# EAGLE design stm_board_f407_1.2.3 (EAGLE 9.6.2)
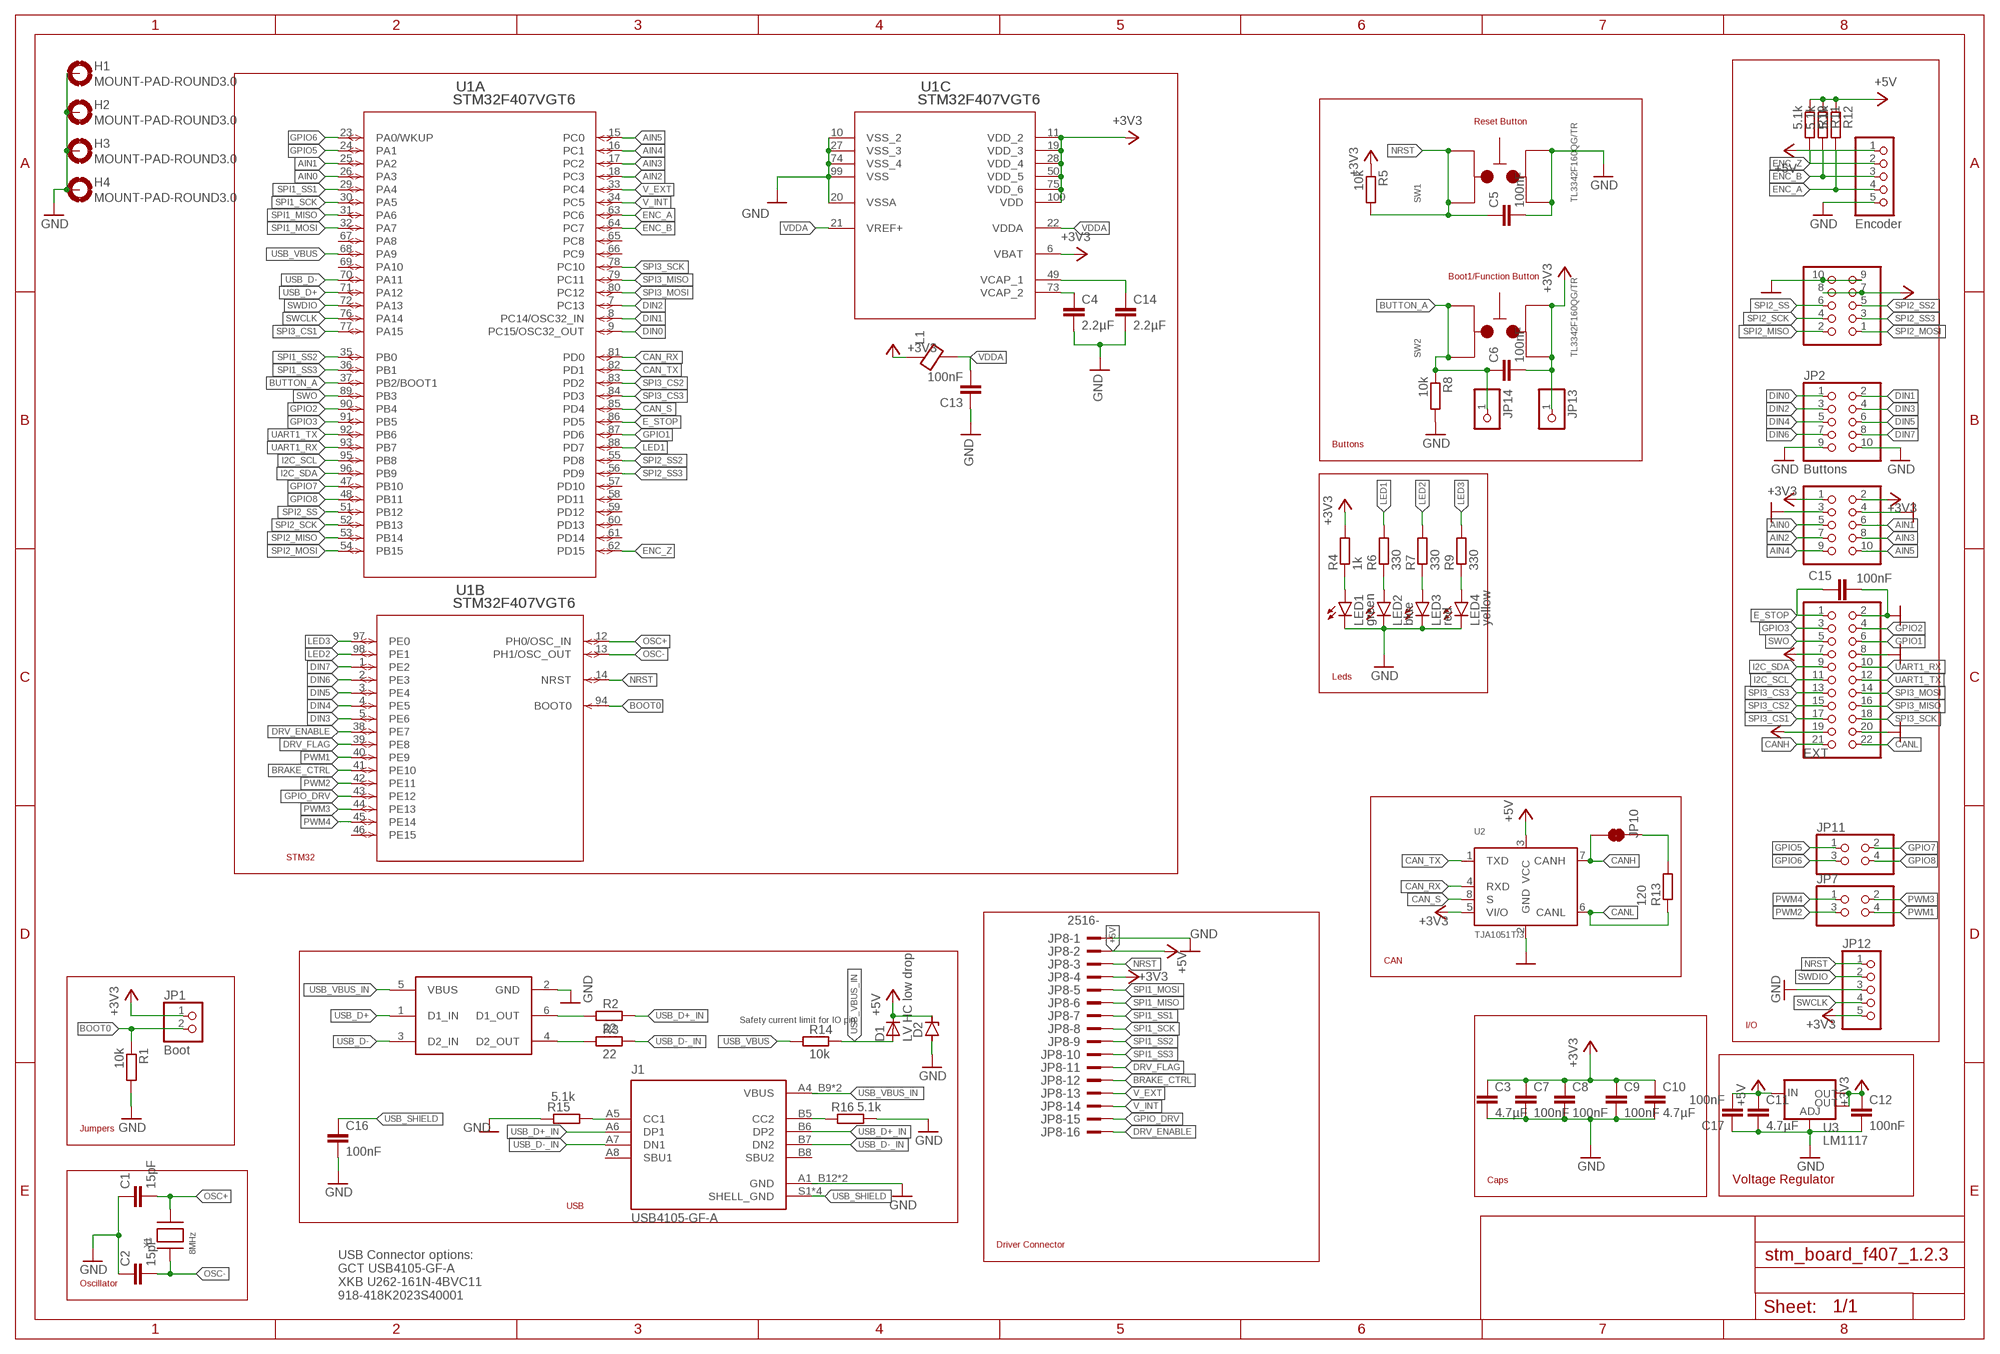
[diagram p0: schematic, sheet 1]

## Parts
C1  15pF  C-EUC0603  [C0603]
C2  15pF  C-EUC0603  [C0603]
C3  4.7µF  C-EUC0805  [C0805]
C4  2.2µF  C-EUC0603  [C0603]
C5  100nF  C-EUC0603  [C0603]
C6  100nF  C-EUC0603  [C0603]
C7  100nF  C-EUC0603  [C0603]
C8  100nF  C-EUC0603  [C0603]
C9  100nF  C-EUC0603  [C0603]
C10  4.7µF  C-EUC0805  [C0805]
C11  4.7µF  C-EUC0805  [C0805]
C12  100nF  C-EUC0603  [C0603]
C13  100nF  C-EUC0603  [C0603]
C14  2.2µF  C-EUC0603  [C0603]
C15  100nF  C-EUC0603  [C0603]
C16  100nF  C-EUC0603  [C0603]
C17  100nF  C-EUC0603  [C0603]
D1  LV HC low drop  DIODESMA  [SMADIODE]
D2  ZENER-DIODESOD80C  [SOD80C]
H1  MOUNT-PAD-ROUND3.0  [3,0-PAD]
H2  MOUNT-PAD-ROUND3.0  [3,0-PAD]
H3  MOUNT-PAD-ROUND3.0  [3,0-PAD]
H4  MOUNT-PAD-ROUND3.0  [3,0-PAD]
J1  USB4105-GF-A  [GCT_USB4105-GF-A]
JP1  Boot  PINHD-1X2  [1X02]
JP2  Buttons  PINHD-2X5  [2X05]
JP3  Analog  PINHD-2X5  [2X05]
JP4  EXT  PINHD-2X11  [2X11]
JP5  Encoder  PINHD-1X5  [1X05]
JP6  SPI  PINHD-2X5  [2X05]
JP7  PINHD-2X2  [2X02]
JP8  2516-  [PAK100/2500-16]
JP10  JUMPER-SMT_2_NC_TRACE_SILK  [SMT-JUMPER_2_NC_TRACE_SILK]
JP11  PINHD-2X2  [2X02]
JP12  PINHD-1X5  [1X05]
JP13  PINHD-1X1  [1X01]
JP14  PINHD-1X1  [1X01]
L1  GZ2012D601TF  BLM21PG331SN1D  [BLM21PG331SN1D]
LED1  green  LEDSML0805  [SML0805]
LED2  blue  LEDSML0805  [SML0805]
LED3  red  LEDSML0805  [SML0805]
LED4  yellow  LEDSML0805  [SML0805]
R1  10k  R-EU_R0603  [R0603]
R2  22  R-EU_R0603  [R0603]
R3  22  R-EU_R0603  [R0603]
R4  1k  R-EU_R0603  [R0603]
R5  10k  R-EU_R0603  [R0603]
R6  330  R-EU_R0603  [R0603]
R7  330  R-EU_R0603  [R0603]
R8  10k  R-EU_R0603  [R0603]
R9  330  R-EU_R0603  [R0603]
R10  5.1k  R-EU_R0603  [R0603]
R11  5.1k  R-EU_R0603  [R0603]
R12  5.1k  R-EU_R0603  [R0603]
R13  120  R-EU_R0603  [R0603]
R14  10k  R-EU_R0603  [R0603]
R15  5.1k  R-EU_R0603  [R0603]
R16  5.1k  R-EU_R0603  [R0603]
SW1  TL3342F160QG/TR  [TL3342F160QG/TR]
SW2  TL3342F160QG/TR  [TL3342F160QG/TR]
U1  STM32F407VGT6  [LQFP100-14X14MM]
U2  TJA1051T/3  [SOT96-1]
U3  LM1117  V_REG_LM1117SOT223  [SOT223]
U4  USBLC6-2SC6  [TSOT-23-6]
X1  8MHz  XTALNX5032  [NX5032]

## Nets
+3V3: C3.1 C6.2 C7.1 C8.1 C9.1 C10.1 C12.1 JP1.1 JP3.1 JP3.2 JP4.7 JP6.7 JP6.8 JP8.4 JP12.5 JP13.1 L1.1 R4.2 R5.1 SW2.1 SW2.2 U1.6(C:VBAT) U1.11(C:VDD_2) U1.19(C:VDD_3) U1.28(C:VDD_4) U1.50(C:VDD_5) U1.75(C:VDD_6) U1.100(C:VDD) U2.5(VI/O) U3.2(OUT) U3.4(OUT)
+5V: C11.1 C17.2 D1.C D2.C JP4.19 JP5.1 JP8.2 R10.1 R11.1 R12.1 U2.3(VCC) U3.3(IN)
AIN0: JP3.5 U1.26(A:PA3)
AIN1: JP3.6 U1.25(A:PA2)
AIN2: JP3.7 U1.18(A:PC3)
AIN3: JP3.8 U1.17(A:PC2)
AIN4: JP3.9 U1.16(A:PC1)
AIN5: JP3.10 U1.15(A:PC0)
BOOT0: JP1.2 R1.1 U1.94(B:BOOT0)
BRAKE_CTRL: JP8.12 U1.41(B:PE10)
BUTTON_A: C6.1 JP14.1 R8.1 SW2.3 SW2.4 U1.37(A:PB2/BOOT1)
CAN_RX: U1.81(A:PD0) U2.4(RXD)
CAN_S: U1.85(A:PD4) U2.8(S)
CAN_TX: U1.82(A:PD1) U2.1(TXD)
CANH: JP4.21 JP10.2 U2.7(CANH)
CANL: JP4.22 R13.1 U2.6(CANL)
DIN0: JP2.1 U1.9(A:PC15/OSC32_OUT)
DIN1: JP2.2 U1.8(A:PC14/OSC32_IN)
DIN2: JP2.3 U1.7(A:PC13)
DIN3: JP2.4 U1.5(B:PE6)
DIN4: JP2.5 U1.4(B:PE5)
DIN5: JP2.6 U1.3(B:PE4)
DIN6: JP2.7 U1.2(B:PE3)
DIN7: JP2.8 U1.1(B:PE2)
DRV_ENABLE: JP8.16 U1.38(B:PE7)
DRV_FLAG: JP8.11 U1.39(B:PE8)
E_STOP: C15.1 JP4.1 U1.86(A:PD5)
ENC_A: JP5.4 R12.2 U1.63(A:PC6)
ENC_B: JP5.3 R11.2 U1.64(A:PC7)
ENC_Z: JP5.2 R10.2 U1.62(A:PD15)
GND: C1.1 C2.1 C3.2 C4.2 C5.2 C7.2 C8.2 C9.2 C10.2 C11.2 C12.2 C13.1 C14.2 C15.2 C16.2 C17.1 D2.A H1.B3,0(MOUNT) H2.B3,0(MOUNT) H3.B3,0(MOUNT) H4.B3,0(MOUNT) J1.A1_B12(GND) J1.B1_A12(GND) JP2.9 JP2.10 JP3.3 JP3.4 JP4.2 JP4.8 JP4.20 JP5.5 JP6.9 JP6.10 JP8.1 JP12.3 LED1.C LED2.C LED3.C LED4.C R1.2 R8.2 R15.1 R16.2 SW1.1 SW1.2 U1.10(C:VSS_2) U1.20(C:VSSA) U1.27(C:VSS_3) U1.74(C:VSS_4) U1.99(C:VSS) U2.2(GND) U3.1(ADJ) U4.2(GND)
GPIO1: JP4.6 U1.87(A:PD6)
GPIO2: JP4.4 U1.90(A:PB4)
GPIO3: JP4.3 U1.91(A:PB5)
GPIO5: JP11.1 U1.24(A:PA1)
GPIO6: JP11.3 U1.23(A:PA0/WKUP)
GPIO7: JP11.2 U1.47(A:PB10)
GPIO8: JP11.4 U1.48(A:PB11)
GPIO_DRV: JP8.15 U1.43(B:PE12)
I2C_SCL: JP4.11 U1.95(A:PB8)
I2C_SDA: JP4.9 U1.96(A:PB9)
LED1: R6.2 U1.88(A:PD7)
LED2: R7.2 U1.98(B:PE1)
LED3: R9.2 U1.97(B:PE0)
N$1: R2.1 U4.6(D1_OUT)
N$2: LED4.A R9.1
N$3: JP10.1 R13.2
N$4: C14.1 U1.49(C:VCAP_1)
N$5: J1.B5(CC2) R16.1
N$6: J1.A5(CC1) R15.2
N$7: C4.1 U1.73(C:VCAP_2)
N$8: R3.1 U4.4(D2_OUT)
N$11: LED1.A R4.1
N$12: LED2.A R6.1
N$13: LED3.A R7.1
NRST: C5.1 JP8.3 JP12.1 R5.2 SW1.3 SW1.4 U1.14(B:NRST)
OSC+: C1.2 U1.12(B:PH0/OSC_IN) X1.P$2
OSC-: C2.2 U1.13(B:PH1/OSC_OUT) X1.P$1
PWM1: JP7.4 U1.40(B:PE9)
PWM2: JP7.3 U1.42(B:PE11)
PWM3: JP7.2 U1.44(B:PE13)
PWM4: JP7.1 U1.45(B:PE14)
SPI1_MISO: JP8.6 U1.31(A:PA6)
SPI1_MOSI: JP8.5 U1.32(A:PA7)
SPI1_SCK: JP8.8 U1.30(A:PA5)
SPI1_SS1: JP8.7 U1.29(A:PA4)
SPI1_SS2: JP8.9 U1.35(A:PB0)
SPI1_SS3: JP8.10 U1.36(A:PB1)
SPI2_MISO: JP6.2 U1.53(A:PB14)
SPI2_MOSI: JP6.1 U1.54(A:PB15)
SPI2_SCK: JP6.4 U1.52(A:PB13)
SPI2_SS: JP6.6 U1.51(A:PB12)
SPI2_SS2: JP6.5 U1.55(A:PD8)
SPI2_SS3: JP6.3 U1.56(A:PD9)
SPI3_CS1: JP4.17 U1.77(A:PA15)
SPI3_CS2: JP4.15 U1.83(A:PD2)
SPI3_CS3: JP4.13 U1.84(A:PD3)
SPI3_MISO: JP4.16 U1.79(A:PC11)
SPI3_MOSI: JP4.14 U1.80(A:PC12)
SPI3_SCK: JP4.18 U1.78(A:PC10)
SWCLK: JP12.4 U1.76(A:PA14)
SWDIO: JP12.2 U1.72(A:PA13)
SWO: JP4.5 U1.89(A:PB3)
UART1_RX: JP4.10 U1.93(A:PB7)
UART1_TX: JP4.12 U1.92(A:PB6)
USB_D+: U1.71(A:PA12) U4.1(D1_IN)
USB_D+_IN: J1.A6(DP1) J1.B6(DP2) R2.2
USB_D-: U1.70(A:PA11) U4.3(D2_IN)
USB_D-_IN: J1.A7(DN1) J1.B7(DN2) R3.2
USB_SHIELD: C16.1 J1.S1(SHELL_GND) J1.S2(SHELL_GND) J1.S3(SHELL_GND) J1.S4(SHELL_GND)
USB_VBUS: R14.1 U1.68(A:PA9)
USB_VBUS_IN: D1.A J1.A4_B9(VBUS) J1.B4_A9(VBUS) R14.2 U4.5(VBUS)
V_EXT: JP8.13 U1.33(A:PC4)
V_INT: JP8.14 U1.34(A:PC5)
VDDA: C13.2 L1.2 U1.21(C:VREF+) U1.22(C:VDDA)
Unconnected: J1.A8(SBU1) J1.B8(SBU2) U1.46(B:PE15) U1.57(A:PD10) U1.58(A:PD11) U1.59(A:PD12) U1.60(A:PD13) U1.61(A:PD14) U1.65(A:PC8) U1.66(A:PC9) U1.67(A:PA8) U1.69(A:PA10)

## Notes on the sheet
- Reset Button
- Boot1/Function Button
- Buttons
- Leds
- STM32
- CAN
- Safety current limit for IO pin
- I/O
- Jumpers
- Caps | Voltage Regulator
- USB
- Driver Connector
- Oscillator
- USB Connector options:
  GCT USB4105-GF-A 
  XKB U262-161N-4BVC11
  918-418K2023S40001

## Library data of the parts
C1-C17 = resistor:C-EU: CAPACITOR, European symbol
D1 = adafruit:DIODE: Diode
D2 = diode:ZENER-DIODE: Z-Diode
H1-H4 = holes:MOUNT-PAD-ROUND: MOUNTING PAD, round
J1 = USB4105-GF-A:USB4105-GF-A: USB-C (USB TYPE-C) USB 2.0 Receptacle Connector 24 (16+8 Dummy) Position Surface Mount, Right Angle; Through Hole Check availability; AVAILABILITY: In Stock; DESCRIPTION: USB-C (USB TYPE-C) USB 2.0 Receptacle Connector 24 (16+8 Dummy) Position Surface Mount, Right Angle; Through Hole; MF: GCT; MP: USB4105-GF-A; PACKAGE: None; PRICE: None; PURCHASE-URL: https://pricing.snapeda.com/search/part/USB4105-GF-A/?ref=eda
JP1 = pinhead:PINHD-1X2: PIN HEADER
JP2 JP3 JP6 = pinhead:PINHD-2X5: PIN HEADER
JP4 = pinhead:PINHD-2X11: PIN HEADER
JP5 JP12 = pinhead:PINHD-1X5: PIN HEADER
JP7 JP11 = pinhead:PINHD-2X2: PIN HEADER
JP8 = con-3m:2516-: 3M (TM) Pak 100 4-Wall Header Source: 3M; OC_FARNELL: unknown; OC_NEWARK: unknown
JP10 = SparkFun-Jumpers:JUMPER-SMT_2_NC_TRACE: Normally closed trace jumper
JP13 JP14 = pinhead:PINHD-1X1: PIN HEADER
L1 = Thermistor_Inductors:BLM21PG331SN1D: FERRITE BEAD 330 OHM 0805 1LN; CREATED_BY: PCBLayout.com; DIGIKEY_PART_NUMBER: 490-5988-2-ND; MANUFACTURER: Murata Electronics North America; MPN: BLM21PG331SN1D; PACKAGE: 0805
LED1-LED4 = led:LED: LED
R1-R16 = resistor:R-EU_: RESISTOR, European symbol
SW1 SW2 = Switch:TL3342F160QG/TR: SWITCH TACTILE SPST-NO 0.05A 12V Manufacturer's datasheet; CREATED_BY: PCBLayout.com; DIGI_KEY_PART_NUMBER: EG2531CT-ND; MANUFACTURER: E-Switch; MPN: TL3342F160QG/TR; PACKAGE: SPST_NO
U1 = STM32:STM32F407VGT6; BUILT_BY: EMA_UL_Team; COPYRIGHT: Copyright (C) 2018 Accelerated Designs. All rights reserved; MANUFACTURER_PART_NUMBER: STM32F407VGT6; SOURCELIBRARY: Updates_to_database_2020-10-19; VENDOR: STMicroelectronics
U2 = TJA1051T_3:TJA1051T/3: High-speed CAN transceiver The TJA1051 is a high-speed CAN transceiver that provides an interface between a Controller Area Network (CAN) protocol controller and the physical two-wire CAN bus. The transceiver is designed for high-speed (up to 1 Mbit/s) CAN applications in the automotive industry,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; AVAILABILITY: Bad; DESCRIPTION: 1/1 Transceiver Half CANbus 8-SO; MF: NXP Semiconductors; MP: TJA1051T/3; PACKAGE: SOIC-8 NXP Semiconductors; PRICE: None
U3 = SparkFun-IC-Power:V_REG_LM1117: Voltage Regulator LM1117 Standard adjustable voltage regulator but in SMD form. Spark Fun Electronics SKU : COM-00595; PROD_ID: VREG-08170
U4 = con_ampusb_10118193-0001LF:USBLC6-2SC6
X1 = adafruit:XTAL: Low cost SMT crystals, no capacitors included

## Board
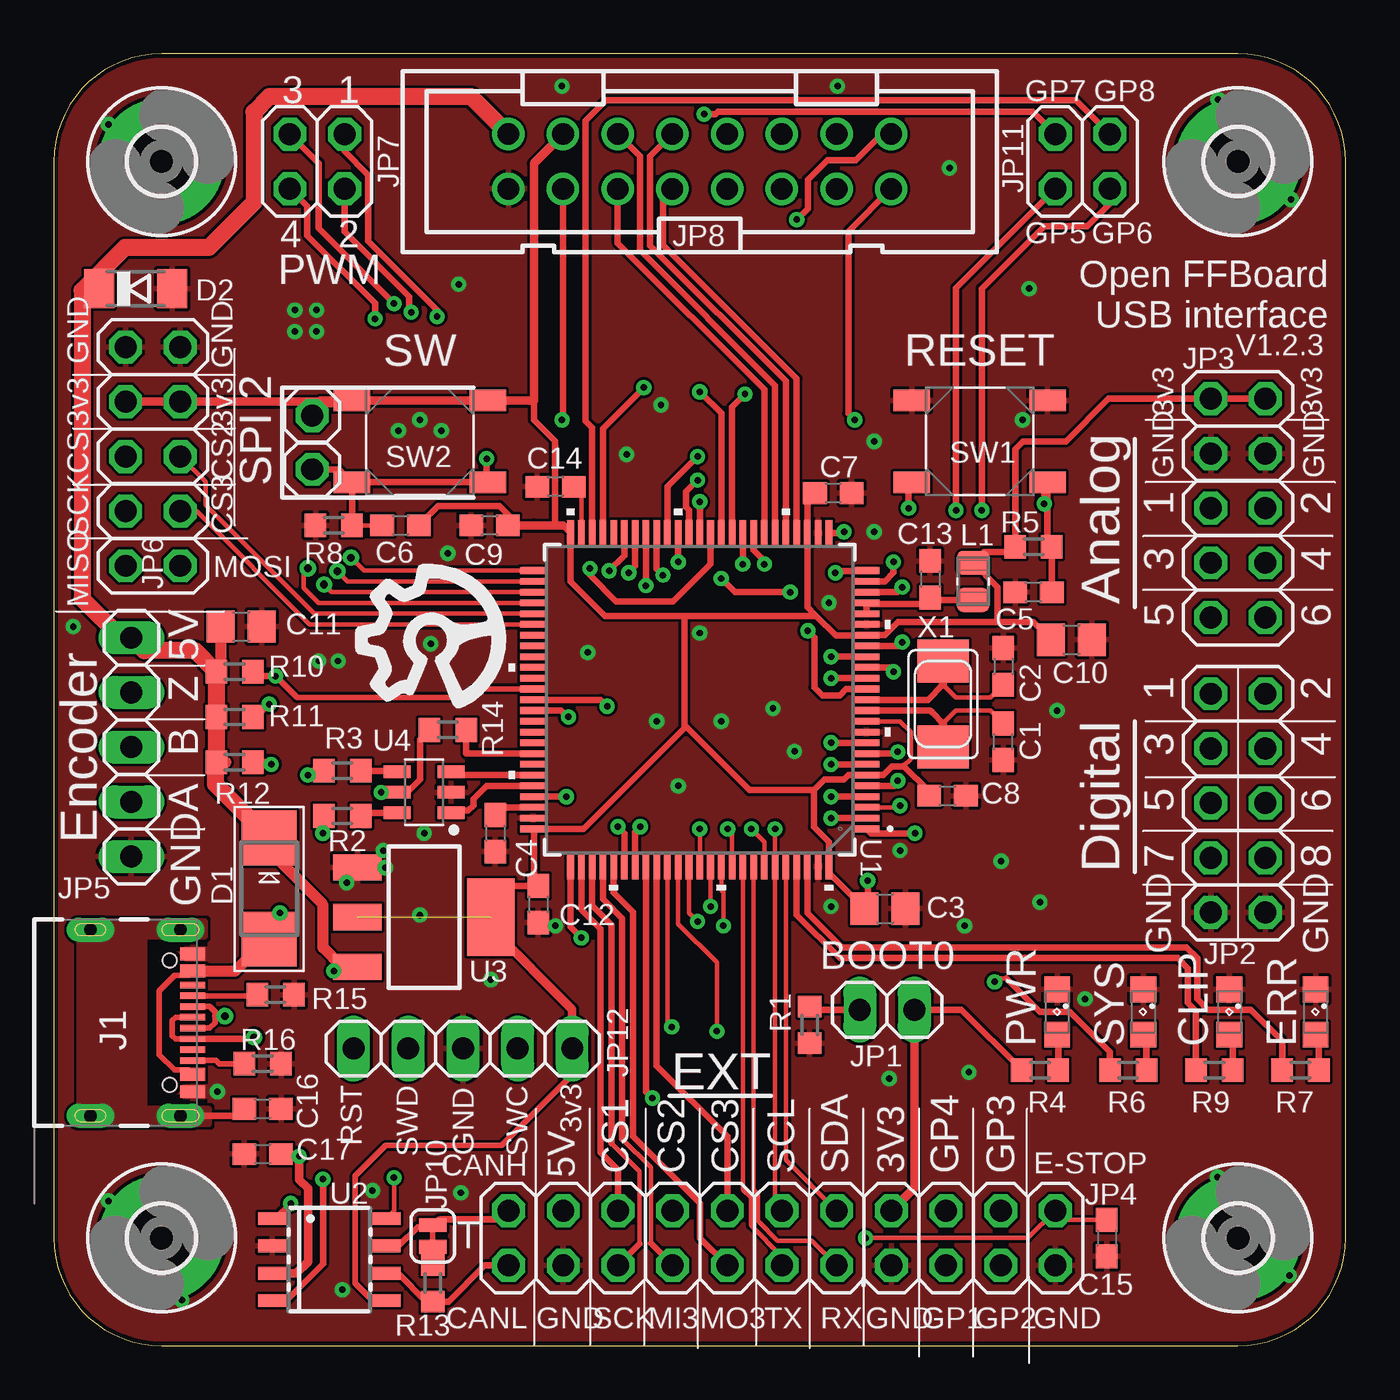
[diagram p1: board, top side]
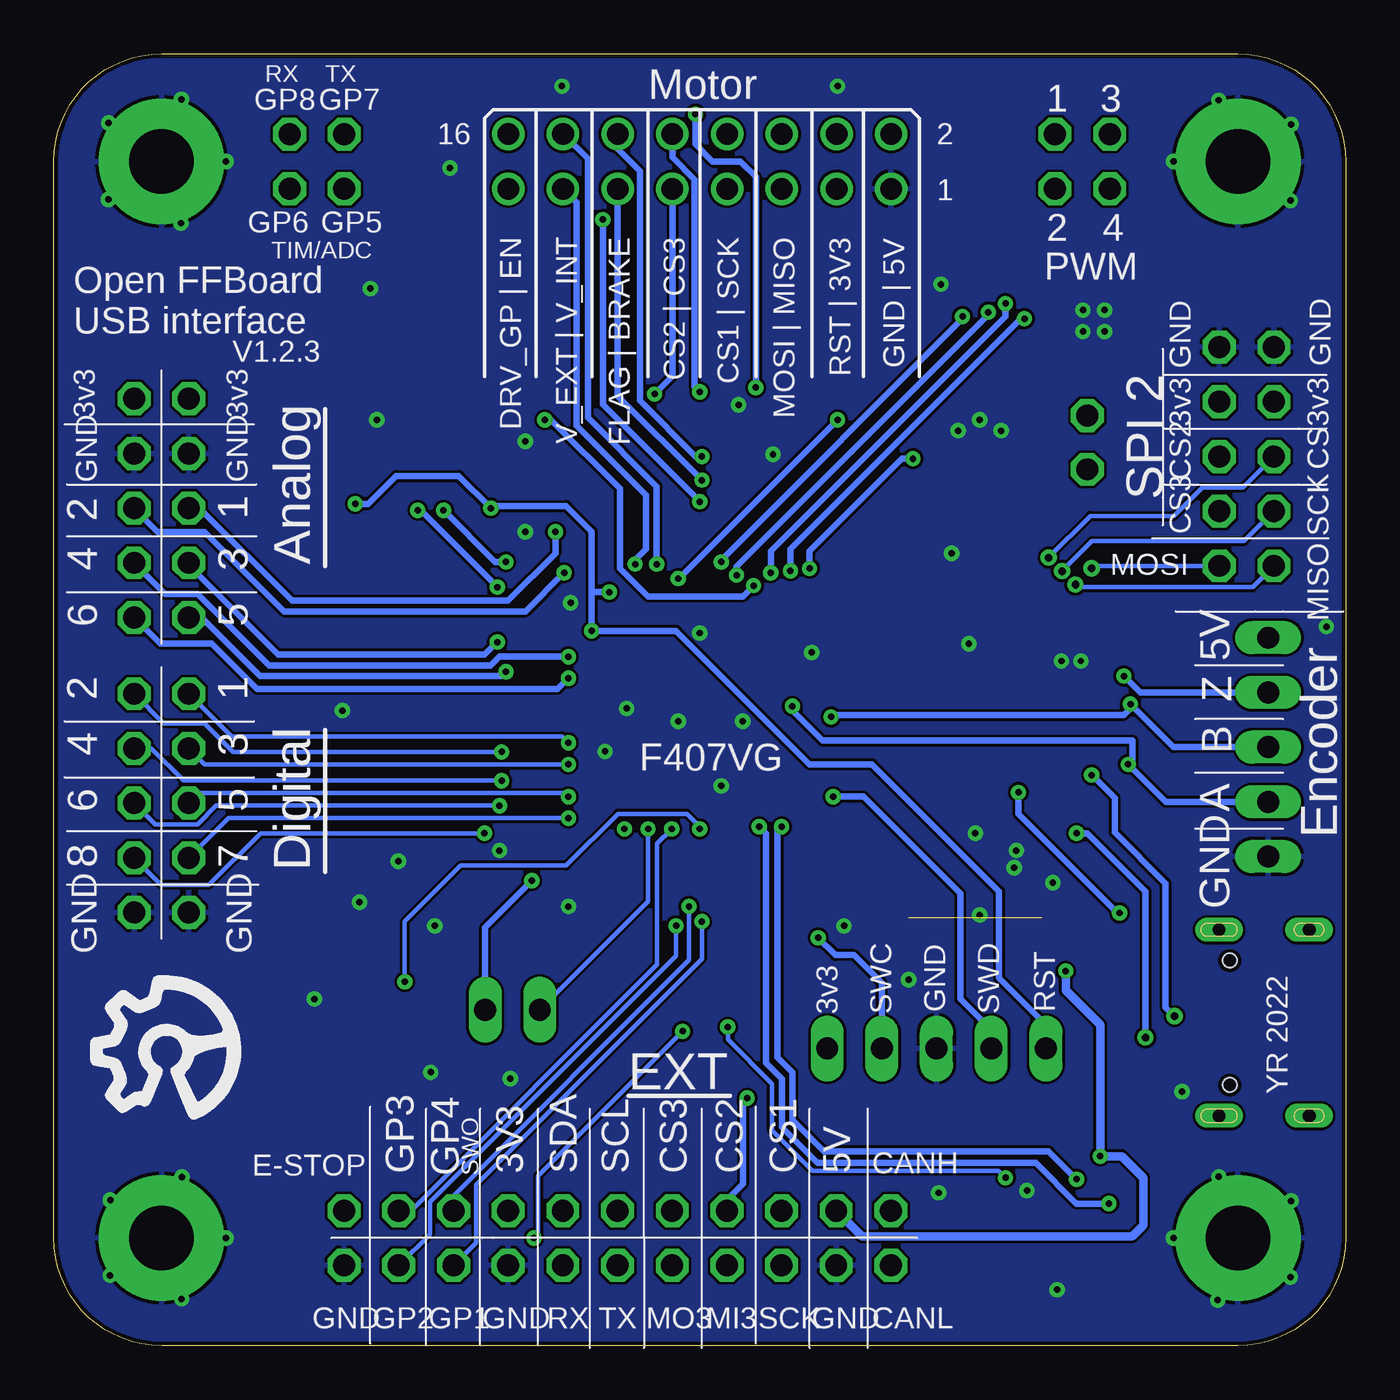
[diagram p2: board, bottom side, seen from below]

Size 60 x 60 mm. Coordinates in mm from the lower left corner, seen from the top.
Outline: 5,0 55,0 arc90 60,5 60,55 arc90 55,60 5,60 arc90 0,55 0,5 arc90 5,0
Copper layers (1*16): Top 0.035mm / dielectric 1.5mm / Bottom 0.035mm
Design rules "jlcpcb *": minimum track width 5mil, minimum drill 0.3mm, track to track 5mil, track to pad 5mil, pad to pad 5mil, via to via 5mil, smd to smd 5mil, copper to edge 0.2mm, drill to drill 8mil, minimum pad ring 10mil, minimum via ring 8mil, stop-mask expansion 2mil, vias tented up to drill 0.4mm, thermal gap 6mil

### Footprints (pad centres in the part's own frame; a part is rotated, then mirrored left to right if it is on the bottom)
C0603 = smd 1.1 x 1: 1 -0.85,0; 2 0.85,0
C0805 = smd 1.3 x 1.5: 1 -0.95,0; 2 0.95,0
SMADIODE = smd 2.54 x 2.54: A 2.349,0; C -2.349,0
SOD80C = smd 1.4 x 1.8: A 1.7,0; C -1.7,0
3,0-PAD = drill 3 pad 5.842: B3,0 0,0
GCT_USB4105-GF-A = smd 0.6 x 1.15: A1_B12 -3.2,4.755; A4_B9 -2.4,4.755; B1_A12 3.2,4.755; B4_A9 2.4,4.755 | smd 0.3 x 1.15: A5 -1.25,4.755; A6 -0.25,4.755; A7 0.25,4.755; A8 1.25,4.755; B5 1.75,4.755; B6 0.75,4.755; B7 -0.75,4.755; B8 -1.75,4.755 | drill 0.6 pad 1.05 long: S1 -4.32,4.18; S4 4.32,4.18 | drill 0.6 pad 1 long: S2 -4.32,0; S3 4.32,0 | hole 0.65: 2.89,3.68; -2.89,3.68
1X02 = drill 1.016 long: 1 -1.27,0; 2 1.27,0
2X05 = drill 1.016 octagon: 1 -5.08,-1.27; 2 -5.08,1.27; 3 -2.54,-1.27; 4 -2.54,1.27; 5 0,-1.27; 6 0,1.27; 7 2.54,-1.27; 8 2.54,1.27; 9 5.08,-1.27; 10 5.08,1.27
2X11 = drill 1.016 octagon: 1 -12.7,-1.27; 2 -12.7,1.27; 3 -10.16,-1.27; 4 -10.16,1.27; 5 -7.62,-1.27; 6 -7.62,1.27; 7 -5.08,-1.27; 8 -5.08,1.27; 9 -2.54,-1.27; 10 -2.54,1.27; 11 0,-1.27; 12 0,1.27; 13 2.54,-1.27; 14 2.54,1.27; 15 5.08,-1.27; 16 5.08,1.27; 17 7.62,-1.27; 18 7.62,1.27; 19 10.16,-1.27; 20 10.16,1.27; 21 12.7,-1.27; 22 12.7,1.27
1X05 = drill 1.016 long: 1 -5.08,0; 2 -2.54,0; 3 0,0; 4 2.54,0; 5 5.08,0
2X02 = drill 1.016 octagon: 1 -1.27,-1.27; 2 -1.27,1.27; 3 1.27,-1.27; 4 1.27,1.27
PAK100/2500-16 = drill 1 pad 1.422: 1 -8.89,-1.27; 2 -8.89,1.27; 3 -6.35,-1.27; 4 -6.35,1.27; 5 -3.81,-1.27; 6 -3.81,1.27; 7 -1.27,-1.27; 8 -1.27,1.27; 9 1.27,-1.27; 10 1.27,1.27; 11 3.81,-1.27; 12 3.81,1.27; 13 6.35,-1.27; 14 6.35,1.27; 15 8.89,-1.27; 16 8.89,1.27
SMT-JUMPER_2_NC_TRACE_SILK = smd 0.635 x 1.27: 1 -0.508,0; 2 0.508,0
1X01 = drill 1.016 octagon: 1 0,0
BLM21PG331SN1D = smd 1.09 x 1.47: 1 -0.865,0; 2 0.865,0
SML0805 = smd 1.2 x 1.2: A 1.05,0; C -1.05,0
R0603 = smd 1 x 1.1: 1 -0.85,0; 2 0.85,0
TL3342F160QG/TR = smd 1.7 x 1: 1 -3.15,-1.9; 2 3.15,-1.9; 3 -3.15,1.9; 4 3.15,1.9
LQFP100-14X14MM = smd 0.305 x 1.194: 1 -6,-7.75; 2 -5.5,-7.75; 3 -5,-7.75; 4 -4.5,-7.75; 5 -4,-7.75; 6 -3.5,-7.75; 7 -3,-7.75; 8 -2.5,-7.75; 9 -2,-7.75; 10 -1.5,-7.75; 11 -1,-7.75; 12 -0.5,-7.75; 13 0,-7.75; 14 0.5,-7.75; 15 1,-7.75; 16 1.5,-7.75; 17 2,-7.75; 18 2.5,-7.75; 19 3,-7.75; 20 3.5,-7.75; 21 4,-7.75; 22 4.5,-7.75; 23 5,-7.75; 24 5.5,-7.75; 25 6,-7.75; 51 6,7.75; 52 5.5,7.75; 53 5,7.75; 54 4.5,7.75; 55 4,7.75; 56 3.5,7.75; 57 3,7.75; 58 2.5,7.75; 59 2,7.75; 60 1.5,7.75; 61 1,7.75; 62 0.5,7.75; 63 0,7.75; 64 -0.5,7.75; 65 -1,7.75; 66 -1.5,7.75; 67 -2,7.75; 68 -2.5,7.75; 69 -3,7.75; 70 -3.5,7.75; 71 -4,7.75; 72 -4.5,7.75; 73 -5,7.75; 74 -5.5,7.75; 75 -6,7.75 | smd 1.194 x 0.305: 26 7.75,-6; 27 7.75,-5.5; 28 7.75,-5; 29 7.75,-4.5; 30 7.75,-4; 31 7.75,-3.5; 32 7.75,-3; 33 7.75,-2.5; 34 7.75,-2; 35 7.75,-1.5; 36 7.75,-1; 37 7.75,-0.5; 38 7.75,0; 39 7.75,0.5; 40 7.75,1; 41 7.75,1.5; 42 7.75,2; 43 7.75,2.5; 44 7.75,3; 45 7.75,3.5; 46 7.75,4; 47 7.75,4.5; 48 7.75,5; 49 7.75,5.5; 50 7.75,6; 76 -7.75,6; 77 -7.75,5.5; 78 -7.75,5; 79 -7.75,4.5; 80 -7.75,4; 81 -7.75,3.5; 82 -7.75,3; 83 -7.75,2.5; 84 -7.75,2; 85 -7.75,1.5; 86 -7.75,1; 87 -7.75,0.5; 88 -7.75,0; 89 -7.75,-0.5; 90 -7.75,-1; 91 -7.75,-1.5; 92 -7.75,-2; 93 -7.75,-2.5; 94 -7.75,-3; 95 -7.75,-3.5; 96 -7.75,-4; 97 -7.75,-4.5; 98 -7.75,-5; 99 -7.75,-5.5; 100 -7.75,-6
SOT96-1 = smd 0.6 x 1.3: 1 -1.905,-2.65; 2 -0.635,-2.65; 3 0.635,-2.65; 4 1.905,-2.65; 5 1.905,2.65; 6 0.635,2.65; 7 -0.635,2.65; 8 -1.905,2.65
SOT223 = smd 1.219 x 2.235: 1 -2.311,-3.099; 2 0,-3.099; 3 2.311,-3.099 | smd 3.6 x 2.2: 4 0,3.099
TSOT-23-6 = smd 1.25 x 0.589: 1 -1.256,0.95; 2 -1.256,0; 3 -1.256,-0.95; 4 1.256,-0.95; 5 1.256,0; 6 1.256,0.95
NX5032 = smd 2 x 2.4: P$1 2,0; P$2 -2,0

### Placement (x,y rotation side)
C1  44.1,28.05 90 top
C2  44.1,31.55 270 top
C3  38.6,20.3 0 top
C4  20.5,23.8 270 top
C5  45.5,35 180 top
C6  16.1,38.1 0 top
C7  36.2,39.6 0 top
C8  41.51,25.54 0 top
C9  20.24,38.1 180 top
C10  47.26,32.79 0 top
C11  8.7,33.4 0 top
C12  22.5,20.5 270 top
C13  40.7,35.6 270 top
C14  23.3,39.9 180 top
C15  48.9,5 270 top
C16  9.7,11 0 top
C17  9.7,8.9 0 top
D1  10,21.23 270 top
D2  3.8,49.1 0 top
H1  55,5 0 top
H2  5,5 0 top
H3  55,55 0 top
H4  5,55 0 top
J1  1.7,15 270 top
JP1  38.7,15.6 180 top
JP2  55,25.2 270 top
JP3  55,38.9 270 top
JP4  33.82,5 180 top
JP5  3.6,27.8 270 top
JP6  4.6,41.3 90 top
JP7  12.23,55 0 top
JP8  30,55 0 top
JP10  17.6,5.1 90 top
JP11  47.78,55 0 top
JP12  19,13.8 0 top
JP13  12,43.2 0 top
JP14  12,40.7 0 top
L1  42.7,35.5 270 top
LED1  46.6,15.5 270 top
LED2  50.6,15.5 270 top
LED3  58.6,15.5 270 top
LED4  54.6,15.5 270 top
R1  35.1,14.9 270 top
R2  13.4,24.6 180 top
R3  13.4,26.7 180 top
R4  45.8,12.8 180 top
R5  45.5,37.1 0 top
R6  49.9,12.8 180 top
R7  57.9,12.8 180 top
R8  13,38.1 180 top
R9  53.9,12.8 180 top
R10  8.4,31.3 0 top
R11  8.4,29.2 0 top
R12  8.4,27.1 0 top
R13  17.6,2.9 90 top
R14  18.3,28.6 180 top
R15  10.3,16.3 180 top
R16  9.7,13.1 0 top
SW1  43,42 180 top
SW2  17,42 180 top
U1  30,30 90 top
U2  12.8,4 270 top
U3  17.2,19.9 270 top
U4  17.2,25.7 180 top
X1  41.3,29.8 90 top

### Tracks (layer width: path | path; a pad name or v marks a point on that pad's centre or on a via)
+3V3  (via drill 0.3)  (1 unrouted)
  Top 0.2: C7.1 35,39.25 | 37.73,32.98 U1.19 | U1.11 39.3,29 39.8,28.5 39.8,27.26 39.47,26.93 39.44,26.9 | C8.1 40.66,25.74
  Top 0.25: U2.5 14.8,2.09 14,2.9 14,7.9 15.4,9.3 20.8,9.3 24.08,12.58 JP12.5
  Top 0.3: JP3.2 JP3.1 48.98,43.98 47,42 45,42 44.65,41.65 R5.1 44.65,36.86 43.2,36.86 L1.1 | U1.75 22.3,24 22.3,21.55 C12.1 21.35,21.35 20.3,20.3 U3.4 | 23.65,38.1 U1.50 | 35,39.25 U1.28 35,34.3 35.4,33.9 | 35.4,33.9 36.32,32.98 37.73,32.98 | 35.3,25.8 35.8,26.3 36.7,26.3 36.9,26.5 U1.6 38.52,26.5 38.92,26.9 39.44,26.9 | 35.3,25.8 35.3,24.1 36,23.4 U1.100 36,21.95 C3.1 37.8,20.45 v37.8,21.6 | 40.66,25.74 39.47,26.93 | 24,36.72 U1.50 | U1.75 24.6,24 29.3,28.7 | 29.3,28.7 29.35,28.75 32.3,25.8 35.3,25.8 | U1.50 24,35.5 25.6,33.9 29.28,33.9 29.29,33.89 | 42.5,36.56 L1.1 | U1.19 38.6,33 39.2,33.6 43.7,33.6 | 43.7,33.6 43.82,33.72 43.82,35.24 L1.1 | 35.4,33.9 29.3,33.9 29.29,33.89 | 29.3,28.7 29.3,33.88 29.29,33.89 | C10.1 45.5,33.6 43.7,33.6 | R4.2 42.15,15.6 JP1.1 | 23.28,38.1 23.28,42.02 22.3,43 22.3,43.9 | C6.2 17.85,39 20.7,39 21.09,38.61 C9.1 | U1.75 22.3,23.95 | JP13.1 12.64,43.84 13.79,43.84
  Top 0.4: JP8.4 22.3,54.92 22.3,43.9 SW2.1 SW2.2 13.79,43.84 JP6.7 JP6.8 | 22.3,38.1 C9.1 23.28,38.1 23.65,38.1 | JP4.7 39.97,7.34 JP1.1 | U3.4 20.3,19.4 24.08,15.62 JP12.5
  Top 0.5: 12.37,43.84 13.79,43.84
  Bottom 0.3: JP1.1 39.97,19.43 v37.8,21.6
+5V  (via drill 0.3)
  Top 0.3: 11.4,8.9 v11.4,8.8 11.3,8.9 C17.2 | U3.3 14.1,17.2
  Top 0.4: U2.3 11.27,3.37 11.8,3.9 11.8,7.3 11.4,7.7 v11.4,8.8 | v13,17.4 13.19,17.59 U3.3
  Top 0.5: R12.1 8,27.1 7.5,26.6 7.46,26.56 | D1.C 10,22.99 12.5,20.49 12.5,18.49 13.4,17.59 U3.3 | D2.C 2.01,49.01 1.31,49.01 | C11.1 7.75,31.5 R10.1
  Top 0.8: R12.1 R11.1 R10.1 6.57,32.28 4.2,32.28 JP5.1 3.12,32.88 1.31,34.69 1.31,49.01 3.3,51 7.2,51 9.3,53.1 9.3,57.3 10.01,58.01 19.37,58.01 JP8.2 | 7.5,26.6 7.5,26.08 D1.C
  Bottom 0.4: JP4.19 | JP4.19 22.47,5.08 9.92,5.08 9.4,5.6 9.4,7.8 10.4,8.8 v11.4,8.8 11.4,14.9 13,16.5 v13,17.4
AIN0  (via drill 0.3)
  Top 0.2: 36.65,37.75 v36.7,37.8
  Top 0.3: U1.26 36.65,37.75
  Bottom 0.3: v36.7,37.8 36.7,36.8 38.9,34.6 48.94,34.6 53.24,38.9 JP3.5
AIN1  (via drill 0.3)
  Top 0.2: 37.73,35.98 U1.25
  Top 0.3: 37.73,35.98 36.56,35.98 36.48,35.9 v36.3,35.9
  Bottom 0.3: JP3.6 55.17,37.8 53,37.8 49.3,34.1 38.1,34.1 v36.3,35.9
AIN2  (via drill 0.3)
  Top 0.3: U1.18 39.22,32.5 v39.4,32.68
  Bottom 0.2: 53.73,36.26 JP3.7
  Bottom 0.3: v39.4,32.68 39.42,32.68 39.99,32.11 49.58,32.11 53.73,36.26
AIN3  (via drill 0.3)
  Top 0.3: U1.17 v36.1,32
  Bottom 0.3: JP3.8 54.82,34.91 53.32,34.91 49.99,31.58 39.72,31.58 39.3,32 v36.1,32
AIN4  (via drill 0.3)
  Top 0.3: v39,31.3 38.8,31.5 U1.16
  Bottom 0.2: JP3.9 53.13,33.82
  Bottom 0.3: 53.13,33.82 50.41,31.1 39.2,31.1 v39,31.3
AIN5  (via drill 0.3)
  Top 0.3: U1.15 v36.1,31
  Bottom 0.3: v36.1,31 36.6,30.5 50.55,30.5 52.67,32.62 55.07,32.62 JP3.10
BOOT0  (via drill 0.3)
  Top 0.2: U1.94 33,23.4 v32.4,24
  Top 0.3: JP1.2 35.25,15.6 R1.1
  Bottom 0.2: v32.4,24 32.4,20.63 JP1.2
BRAKE_CTRL  (via drill 0.3)
  Top 0.3: U1.41 28.5,39.9 v29.9,41.3
  Bottom 0.3: v29.9,41.3 30.19,41.3 32.78,43.89 32.78,54.56 33.81,55.59 JP8.12
BUTTON_A  (via drill 0.3)
  Top 0.2: C6.1 R8.1
  Top 0.3: v24.9,36.1 24.9,35.79 26.12,34.57 28.76,34.57 30.5,36.31 U1.37 | v20.1,41.2 20.1,40.15 SW2.3 SW2.4 | SW2.4 R8.1 | JP14.1 13.25,40.7 SW2.4
  Bottom 0.3: v24.9,36.1 24.9,36.9 20.6,41.2 v20.1,41.2
CAN_RX  (via drill 0.3)
  Top 0.3: v26.2,24.1 26.5,23.8 U1.81 | U2.4 10.8,2.09 12.5,3.8 v12.5,7.73
  Bottom 0.3: v26.2,24.1 26.4,23.9 26.4,13.4 25.7,12.7 25.7,10.5 24.23,9.03 13.8,9.03 v12.5,7.73
CAN_S  (via drill 0.3)
  Top 0.2: U2.8 15.8,6.26 v15.8,7.8 | U1.85 28.5,15 v28.7,14.8
  Bottom 0.2: v15.8,7.8 16.12,8.12 24.76,8.12 26.64,10 26.64,12.16 28.7,14.22 v28.7,14.8
CAN_TX  (via drill 0.3)
  Top 0.3: v11,6.6 10.3,5.91 U2.1 | v27.23,24.1 27,23.87 U1.82
  Bottom 0.3: v11,6.6 12.5,6.6 14.4,8.5 24.54,8.5 26.18,10.14 26.18,12.38 26.93,13.13 26.93,23.8 v27.23,24.1
CANH
  Top 0.25: 16.89,5.51 17.5,5.51 JP10.2 17.86,5.87 17.96,5.87
  Top 0.3: U2.7 16.02,4.63 16.89,5.51 17.6,5.51 17.96,5.87 20.71,5.87 JP4.21
CANL
  Top 0.3: U2.6 15.98,3.37 17.3,2.05 R13.1 18.33,2.05 20.01,3.73 JP4.22
DIN0  (via drill 0.3)
  Top 0.3: v36.1,28 U1.9
  Bottom 0.2: JP2.1 51.75,28.3 36.4,28.3 v36.1,28
DIN1  (via drill 0.3)
  Top 0.2: 39.12,27.5 v39.2,27.58
  Top 0.3: U1.8 39.12,27.5
  Bottom 0.2: v39.2,27.58 51.68,27.58 53,28.9 54.89,28.9 JP2.2
DIN2  (via drill 0.3)
  Top 0.3: v36.1,27 U1.7
  Bottom 0.2: JP2.3 52.99,27 v36.1,27
DIN3  (via drill 0.3)
  Top 0.2: 39.2,26.18 v39.2,26.24
  Top 0.3: 39.2,26.18 39.02,26 U1.5
  Bottom 0.2: v39.2,26.24 53.97,26.24 55.47,27.74 JP2.4
DIN4  (via drill 0.3)
  Top 0.3: v36.1,25.5 U1.4
  Bottom 0.2: v36.1,25.5 36.26,25.66 53.27,25.66 JP2.5
DIN5  (via drill 0.3)
  Top 0.2: U1.3 39.22,25 v39.3,25.08
  Bottom 0.2: v39.3,25.08 52.45,25.08 53.32,24.21 55.28,24.21 JP2.6
DIN6  (via drill 0.3)
  Top 0.3: v36.1,24.5 U1.2
  Bottom 0.2: JP2.7 51.89,24.5 v36.1,24.5
DIN7  (via drill 0.3)
  Top 0.3: v40,23.8 37.95,23.8 U1.1
  Bottom 0.2: v40,23.8 50.4,23.8 52.8,21.4 55.01,21.4 JP2.8
DRV_ENABLE  (via drill 0.3)
  Top 0.3: U1.38 v30,39.2 | JP8.16 38.47,56.27 37.26,55.06 35.92,55.06 35.02,54.16 35.02,52.82 v34.5,52.3
  Bottom 0.3: v30,39.2 34.5,43.7 v34.5,52.3
DRV_FLAG  (via drill 0.3)
  Top 0.3: U1.39 29.5,38.81 29.37,38.94 29.37,39.67 v29.9,40.2
  Bottom 0.3: v29.9,40.2 33.81,44.11 JP8.11
E_STOP  (via drill 0.3)
  Top 0.2: U1.86 29,19.6 30.8,17.8 v30.8,14.6 | v37.7,5 45.25,5 JP4.1 46.94,5.85 C15.1
  Bottom 0.2: v30.8,14.6 37.5,7.9 37.5,5.2 v37.7,5
ENC_A  (via drill 0.3)
  Top 0.3: U1.63 25.4,30 v25.7,29.7 | v10.1,27 10,27.1 R12.2
  Bottom 0.3: JP5.4 8.36,25.26 v10.1,27 9.9,27.2 9.9,28.1 24.3,28.1 25.7,29.5 v25.7,29.7
ENC_B  (via drill 0.3)
  Top 0.3: U1.64 23.55,29.5 23.85,29.2 v23.9,29.2 | v10,29.8 9.4,29.2 R11.2
  Bottom 0.3: v23.9,29.2 23.8,29.3 10.3,29.3 9.8,29.8 v10,29.8 8,27.8 JP5.3
ENC_Z  (via drill 0.3)
  Top 0.254: U1.62 19.5,30.5 19.1,30.1 11.3,30.1 v10.3,31.1
  Top 0.3: 9.45,31.5 R10.2 9.45,31.1 v10.3,31.1
  Bottom 0.3: JP5.2 9.54,30.34 v10.3,31.1
GND  (via drill 0.3)
  other vias: 45,43 17,43 20.3,17 15.4,22.2 18.8,49.3 23.6,58.5 36.4,58.5 36.1,20.4 15.3,23 28.2,43.7 26.6,41.4 52,5 54.05,7.84 57.38,6.76 57.39,3.27 54.06,2.18 52,55 54.08,57.88 57.45,56.79 57.46,53.24 54.09,52.14 8,55 2.57,53.18 2.54,56.72 5.89,57.85 8,5 5.94,2.12 2.57,3.18 2.54,6.72 5.89,7.85 39.3,23 36,34.5 28,29 31,29 29,26 47.9,16.1 24.8,32.2 33.4,29.6 12.2,47.1 13.2,31.8 13.4,2.6 42.5,12.7 45.8,20.6 46.6,29.5 38.1,37.8 38.1,42 41.6,54.7 45.3,49.1 18.3,36.8 17.5,32.6 12.3,31.8 23.3,19.5 38.8,12.4 14.8,7.2 0.9,33.4 34.4,27.6 30,33.1 12.2,48.1 11.2,48.1 11.2,47.1 16,42.5 18,42.5 44,22.5 18.9,7.1 13.6,21.5 17.2,23.8 7.6,11.8 42.3,19.5 17,20
  pour Top (rank 5): -1,61 -1,-1 61,-1 61,61
  pour Bottom: -2,61 -2,-1 60,-1 60,61
  pour Top (no thermals): 6.1,17.9 8.2,17.9 8.2,18.5 6.1,18.5
  pour Top (no thermals): 6,11.5 8.1,11.5 8.1,12.1 6,12.1
GPIO1  (via drill 0.3)
  Top 0.2: U1.87 29.5,20.1 v29.9,19.7
  Bottom 0.2: v29.9,19.7 29.9,17.97 40.39,7.48 40.39,4.78 JP4.6
GPIO2  (via drill 0.3)
  Top 0.2: U1.90 31,21.15 31.1,21.05 v31.1,19.5
  Bottom 0.2: JP4.4 42.53,5.18 42.53,6.68 31.1,18.11 v31.1,19.5
GPIO3  (via drill 0.3)
  Top 0.2: U1.91 31.5,23.8 v31.3,24
  Bottom 0.2: v31.3,24 31.98,23.32 31.98,17.7 43.41,6.27 JP4.3
GPIO5  (via drill 0.3)
  Top 0.3: U1.24 38.6,35.5 39,35.9 v39,36.4 | JP11.1 41.9,49.12 v41.9,38.8
  Bottom 0.3: v41.9,38.8 39.5,36.4 v39,36.4
GPIO6  (via drill 0.3)
  Top 0.3: U1.23 39.17,35 v39.4,35.23 | v43.1,38.8 43.1,49.1 46,52 48,52 49.05,53.05 JP11.3
  Bottom 0.3: v39.4,35.23 42.97,38.8 v43.1,38.8
GPIO7  (via drill 0.3)
  Top 0.3: JP11.2 45.48,57.3 30.84,57.3 30.74,57.2 v30.2,57.2 | v27.4,44.5 25.5,42.6 U1.47
  Bottom 0.3: v30.2,57.2 30.2,55.8 29.4,55 28.1,55 27.4,54.3 v27.4,44.5
GPIO8
  Top 0.3: U1.48 25,42.65 24.7,42.95 24.7,56.9 25.66,57.85 47.47,57.85 JP11.4
GPIO_DRV  (via drill 0.3)
  Top 0.3: U1.43 v27.5,35.3 | v37.2,43 36.9,43.3 36.9,51.74 JP8.15
  Bottom 0.3: v27.5,35.3 28,34.8 32.4,34.8 33.7,36.1 33.7,39.8 36.9,43 v37.2,43
I2C_SCL  (via drill 0.3)
  Top 0.2: v33.5,24 U1.95 33.5,6.59 JP4.11
I2C_SDA
  Top 0.2: U1.96 34,8.63 JP4.9
LED1  (via drill 0.3)
  Top 0.2: U1.88 v30,24 | 44.25,17.05 43.85,17.05 v43.7,16.9
  Top 0.3: R6.2 49.05,13.65 47.2,15.5 45.8,15.5 44.25,17.05
  Bottom 0.2: v30,24 30,24.1 30.6,24.7 33.8,24.7 36.2,22.3 41.1,22.3 43.7,19.7 v43.7,16.9
LED2
  Top 0.3: R7.2 57.05,14.15 55.6,15.6 53.6,15.6 53.1,16.1 53.1,18 52.6,18.5 36.61,18.5 35,20.11 U1.98
LED3
  Top 0.3: U1.97 34.5,20.01 36.51,18 52.2,18 52.67,17.53 52.67,15.92 53.05,15.55 R9.2
N$1
  Top 0.3: R2.1 14.4,24.75 U4.6
N$2
  Top 0.2: LED4.A 54.75,14.45
  Top 0.3: R9.1 54.75,14.45
N$3
  Top 0.25: JP10.1 17.6,4
  Top 0.3: R13.2 17.6,4 17.6,4.69
N$4
  Top 0.2: U1.49 24.5,39.55 C14.1
N$5
  Top 0.254: J1.B5 7.54,13.25 7.69,13.1 R16.1
N$6
  Top 0.254: J1.A5 9.4,16.25 R15.2
N$7
  Top 0.2: 20.85,25 C4.1
  Top 0.3: U1.73 20.85,25
N$8
  Top 0.3: R3.1 15.89,26.7 U4.4
N$11
  Top 0.2: LED1.A 46.65,14.4
  Top 0.3: R4.1 46.65,14.4
N$12
  Top 0.2: LED2.A 50.75,14.3
  Top 0.3: R6.1 50.75,14.3
N$13
  Top 0.2: LED3.A 58.75,14.3
  Top 0.3: R7.1 58.75,14.3
NRST  (via drill 0.3)
  Top 0.2: 39.7,39.95 SW1.4 40.35,40.1
  Top 0.3: U1.14 36.8,30.5 36.5,30.2 35.7,30.2 35.32,30.58 35.32,32.9 v35.02,33.2 | v39.7,38.9 39.7,39.95 | C5.1 R5.2 46.15,37.3 SW1.3 46,39.95 v46,39.1 | JP8.3 23.65,43.05 v23.6,43 | v31,35.63 31.63,35 v34.2,35
  Bottom 0.3: 35.02,35 35.02,37.82 36.2,39 39.6,39 v39.7,38.9 41.2,40.4 44.1,40.4 45.4,39.1 v46,39.1 | 35.02,35 v35.02,33.2 31.1,33.2 24.9,27 22,27 16.1,21.1 16.1,17.08 13.92,14.9 JP12.1 | v31,35.63 30.97,35.63 v23.6,43 | v34.2,35 35.02,35
OSC+
  Top 0.2: C1.2 43.5,29.5 41.9,29.5 41.3,28.9
  Top 0.3: 41.3,28.9 40.8,29.4 40.7,29.5 U1.12
  Top 0.4: X1.P$2 41.3,28.9
OSC-
  Top 0.2: C2.2 43.5,30.1 41.9,30.1 41.3,30.7
  Top 0.3: U1.13 40.6,30 41.3,30.7
  Top 0.4: X1.P$1 41.3,30.7
PWM1  (via drill 0.3)
  Top 0.3: JP7.4 13.5,55.47 14.6,54.37 14.6,51.3 17.8,48.1 v17.8,47.8 | v29,36.4 U1.40
  Bottom 0.3: v17.8,47.8 17.8,47.7 29,36.5 v29,36.4
PWM2  (via drill 0.3)
  Top 0.2: v16.6,48 16.5,48.1
  Top 0.3: U1.42 28,36.08 v28.29,35.79 | 16.5,48.1 16.5,48.73 13.5,51.73 JP7.3
  Bottom 0.2: 16.6,47.88 v16.6,48
  Bottom 0.3: v28.29,35.79 28.29,36.19 16.6,47.88
PWM3  (via drill 0.3)
  Top 0.3: JP7.2 12.3,54.93 12.3,51.9 v15.8,48.4 | U1.44 27,36.2 v26.7,35.9
  Bottom 0.3: v15.8,48.4 15.8,47.8 22.8,40.8 26.7,36.9 v26.7,35.9
PWM4  (via drill 0.3)
  Top 0.3: U1.45 26.5,36.7 v25.79,35.99 | v14.92,47.7 14.92,48.42 11.77,51.56 11.77,52.92 JP7.1
  Bottom 0.3: v25.79,35.99 25.79,36.99 15.08,47.7 v14.92,47.7
SPI1_MISO
  Top 0.3: U1.31 33.5,44.6 27.22,50.88 27.22,55.24 JP8.6
SPI1_MOSI
  Top 0.3: U1.32 33,44.4 26.19,51.21 JP8.5
SPI1_SCK
  Top 0.3: U1.30 34,44.8 27.7,51.1 27.7,55.24 JP8.8
SPI1_SS1
  Top 0.3: U1.29 34.5,44.9 28.3,51.1 28.3,53.3 JP8.7
SPI1_SS2  (via drill 0.3)
  Top 0.3: v32.1,44.2 31.5,43.6 U1.35
  Bottom 0.3: JP8.9 31.27,45.03 v32.1,44.2
SPI1_SS3  (via drill 0.3)
  Top 0.3: v30,44.3 v30.01,44.3 31,43.31 U1.36
  Bottom 0.3: JP8.10 31.27,55.19 30.24,54.16 30.24,44.54 v30,44.3
SPI2_MISO  (via drill 0.35)
  Top 0.2: v12.55,35.35 12.9,35 U1.53
  Bottom 0.2: v12.55,35.35 12.43,35.23 4.32,35.23 JP6.2
SPI2_MOSI  (via drill 0.35)
  Top 0.2: U1.54 12.3,34.5 11.6,35.2 11.6,35.9 v11.8,36.1
  Bottom 0.2: JP6.1 11.68,36.22 v11.8,36.1
SPI2_SCK  (via drill 0.35)
  Top 0.2: v13.18,35.98 13.65,35.5 U1.52
  Bottom 0.2: JP6.4 4.73,37.36 11.79,37.36 v13.18,35.98
SPI2_SS  (via drill 0.35)
  Top 0.2: v13.8,36.6 14.4,36 U1.51
  Bottom 0.2: JP6.6 4.77,39.86 6.66,39.86 7.98,38.54 11.86,38.54 v13.8,36.6
SPI2_SS2
  Top 0.2: U1.55 12.09,34 7.05,39.05 7.05,40.12 JP6.5
SPI2_SS3
  Top 0.2: U1.56 11.89,33.5 6.63,38.76 JP6.3
SPI3_CS1
  Top 0.3: JP4.17 26.2,8.17 25.4,8.97 25.4,19.35 24.5,20.25 U1.77
SPI3_CS2  (via drill 0.3)
  Top 0.3: U1.83 27.5,11.8 v27.8,11.5
  Bottom 0.3: v27.8,11.5 28,11.3 28,7.51 28.74,6.77 JP4.15
SPI3_CS3
  Top 0.3: U1.84 28,13 31.28,9.72 JP4.13
SPI3_MISO
  Top 0.2: 27.73,4.74 27.73,8.28 26.4,9.6
  Top 0.3: U1.79 25.5,20.75 26.4,19.85 26.4,9.6 | JP4.16 27.73,4.74
SPI3_MOSI
  Top 0.3: U1.80 26,21.05 26.9,20.15 26.9,9.73 30.02,6.62 30.02,4.99 JP4.14
SPI3_SCK
  Top 0.2: 25.9,9.4 27.2,8.1 27.2,4.73
  Top 0.3: U1.78 25,20.45 25.9,19.55 25.9,9.4 | 27.2,4.73 JP4.18
SWCLK  (via drill 0.3)
  Top 0.3: U1.76 24,19.45 v24.5,18.95
  Bottom 0.3: v24.5,18.95 23.7,18.15 22.84,18.15 21.54,16.84 JP12.4
SWDIO  (via drill 0.3)
  Top 0.3: U1.72 v23.8,25.5
  Bottom 0.3: v23.8,25.5 22.4,25.5 17.9,21 17.9,16.1 16.46,14.66 JP12.2
SWO  (via drill 0.3)
  Top 0.2: U1.89 v30.5,20.4
  Bottom 0.2: v30.5,20.4 30.5,17.91 41.44,6.97 JP4.5
UART1_RX
  Top 0.2: JP4.10 35.21,4.88 33.61,4.88 32.7,5.79 32.7,7.05 32.5,7.25 U1.93
UART1_TX
  Top 0.2: JP4.12 33.82,4.13 32.37,5.58 32.37,6.88 32,7.25 U1.92
USB_D+
  Top 0.3: U4.1 18.56,24.85 19.25,24.85 19.5,25.1 19.5,25.4 20.1,26 U1.71
USB_D+_IN  (via drill 0.3, 0.35)
  Top 0.254: J1.B6 5.65,14.25 5.5,14.4 5.5,15.1 5.65,15.25 J1.A6
  Top 0.3: R2.2 12.5,24.6 v12.5,23.8 | v9.3,14.32 9.23,14.25 J1.B6
  Bottom 0.3: v12.5,23.8 12,23.8 9.3,21.1 v9.3,14.32
USB_D-
  Top 0.3: U1.70 18.61,26.5 U4.3
USB_D-_IN  (via drill 0.3, 0.35)
  Top 0.254: J1.B7 7.24,15.75 7.48,15.51 7.48,15.3 7.48,14.99 7.24,14.75 J1.A7
  Top 0.3: v11.8,26.5 11.99,26.7 R3.2 | v7.95,15.3 7.48,15.3
  Bottom 0.3: v11.8,26.5 10.73,25.44 10.73,23.84 8.37,21.47 8.37,15.72 v7.95,15.3
USB_SHIELD
  Top 0.3: C16.1 8.53,10.68 J1.S4
  pour Top (no thermals): 7,19 4.2,19 4.2,11 7.2,11 7.2,10.3 1.2,10.3 1.2,19.7 7,19.7
USB_VBUS
  Top 0.3: U1.68 19.15,27.5 R14.1
USB_VBUS_IN  (via drill 0.3)
  Top 0.254: J1.B4_A9 6.25,12.8 5.61,12.8 4.9,13.51 4.9,16.49 5.61,17.2 6.25,17.2 J1.A4_B9
  Top 0.3: R14.2 17,28.15 17,26.3 16.4,25.7 v15.2,25.7 | v10.5,20.1 10.5,19.38 D1.A
  Top 0.4: D1.A 10,18.52 | U4.5 v15.2,25.7
  Top 0.5: D1.A 9.9,18.88 8.42,17.4 J1.A4_B9
  Bottom 0.3: v15.2,25.7 15.2,24.69 10.61,20.1 v10.5,20.1
V_EXT  (via drill 0.3)
  Top 0.3: v33,36.3 33,36.45 32.5,36.95 U1.33
  Bottom 0.3: JP8.13 35.73,53.11 35.73,42.74 32.5,39.51 32.5,37 33,36.5 v33,36.3
V_INT  (via drill 0.3)
  Top 0.3: U1.34 v32,36.3
  Bottom 0.3: v32,36.3 32,39.9 35.2,43.1 35.2,55.12 JP8.14
VDDA
  Top 0.2: U1.21 U1.22 | C13.2 40.4,34.45 | 37.8,34.45 37.75,34.4
  Top 0.3: 40.4,34.45 37.8,34.45 | U1.21 37.75,34.4 | C13.2 40.81,34.64 L1.2

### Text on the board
tPlace: 3 | 1 | GP7 | GP8 | 4 | 2 | GP5 | GP6 | Open FFBoard / USB interface | PWM | V1.2.3 | GND | SW | RESET | GND | SPI 2 | 3v3 | 3v3 | 3v3 | 3v3 | CS | CS2 | GND | GND | 1 | 2 | SCK | CS3 | Analog | MOSI | 3 | 4 | MISO | 5 | 6 | Encoder | 5V | Z | 1 | 2 | B | 3 | 4 | Digital | A | 5 | 6 | 7 | 8 | GND | BOOT0 | GND | GND | PWR | SYS | CLIP | ERR | RST | SWD | GND | SWC | 3v3 | EXT | CANH | 5V | CS1 | CS2 | CS3 | SCL | SDA | 3V3 | GP4 | GP3 | E-STOP | T | CANL | GND | SCK | MI3 | MO3 | TX | RX | GND | GP1 | GP2 | GND
bPlace: TX | RX | Motor | 3 | 1 | GP7 | GP8 | 2 | 16 | 1 | RST | 3V3 | MOSI | MISO | CS1 | SCK | CS2 | CS3 | FLAG | BRAKE | V_EXT | V_INT | DRV_GP | EN | GP5 | GP6 | 4 | 2 | GND | 5V | PWM | TIM/ADC | V1.2.3 | Open FFBoard / USB interface | GND | GND | 3v3 | 3v3 | 3v3 | 3v3 | CS | CS2 | Analog | GND | GND | SPI 2 | SCK | CS3 | 1 | 2 | MISO | MOSI | 3 | 4 | 5 | 6 | 5V | Z | 1 | 2 | B | F407VG | 3 | 4 | A | Digital | 5 | 6 | Encoder | 7 | 8 | GND | GND | GND | RST | GND | SWD | SWC | 3v3 | YR 2022 | EXT | E-STOP | CANH | 5V | CS1 | CS2 | CS3 | SCL | SDA | 3V3 | SWO | GP4 | GP3 | CANL | GND | SCK | MI3 | MO3 | TX | RX | GND | GP1 | GP2 | GND

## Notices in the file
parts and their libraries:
SparkFun-IC-Power: Licensing: Creative Commons ShareAlike 4.0 International - https://creativecommons.org/licenses/by-sa/4.0
